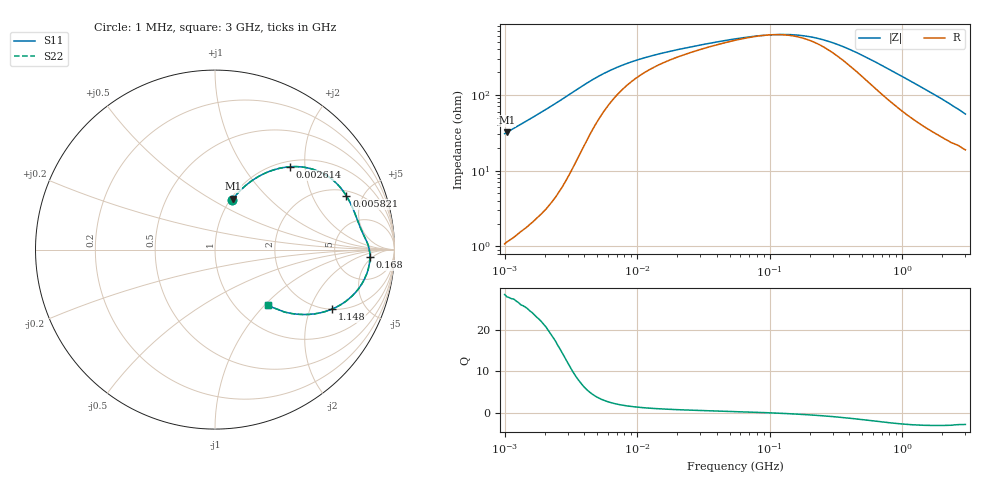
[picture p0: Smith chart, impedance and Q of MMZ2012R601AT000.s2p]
! S-parameter Generated by TDK Corporation
! Copyright(C) 2016 TDK Corporation.
! All Rights Reserved.
! TDK P/N: MMZ2012R601AT000 (Chip Beads)
! Property: |Z|=600¶ at 100MHz
! Size(LxWxT): 2x1.25x0.85mm, 0.079x0.049x0.033inches
! Model Type: s2p (Touchstone File Format Version 1.0)
! Frequency: DC=Yes Start=1MHz Stop=3000MHz 202points Log-sweep
! Note: This model was converted from impedance.
! Model Generated on May. 16, 2016
! Hash(MD5):
! Port Assignments:
!  1 ---@@@--- 2
! Applicable Conditions:
!  Temperature = 25 degC
!  DC Bias Current = 0 A
!  Small Signal Operation
! Terms and conditions regarding TDK Simulation Models
! (1)This simulation model is being provided solely for informational purposes. Please refer to the specifications of the products in terms of detailed characteristics of such products.
! (2)In no event shall TDK Corporation of any of its subsidiaries be liable for any loss or damage arising, directly or indirectly,
!  From any information contained in this simulation model, including, but not limited to loss or damages arising from any inaccuracies, omissions or errors in connection with such information.
! (3)Any and all copyrights on this simulation model are owned by TDK Corporation.
!  Duplication or redistribution of this simulation model without prior written permission from TDK Corporation is prohibited.
! (4)This simulation model is subject to any modification or change without any prior notice.
! (5)Neither TDK Corporation nor any of its subsidiaries shall make any warranty, express or implied,
!  Including but not limited to the correctness, implied warranties of merchantability and fitness for a particular purpose with respect to this simulation models.
! (6)The use of this simulation model shall be deemed to have consented to the terms and conditions hereof.
# MHz S MA R 50
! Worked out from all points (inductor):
!   201 points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, 1 MHz to 3 GHz, reference 50 ohm
!   read as one part in series: L = 4.88 uH near 1.041 MHz
!   highest Q = 27.9 at 1.041 MHz (marker M1), where L = 4.87 uH
!   self-resonance near 99.71 MHz
!   S11 on the Smith chart (normalised r, x): 1 MHz: 1.02, +0.61; 2.614 MHz: 1.11, +1.67; 5.821 MHz: 2.32, +3.71; 168 MHz: 12, -4; 1.148 GHz: 2.01, -2.87; 3 GHz: 1.37, -1.05
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1  0.2901 71.1  0.9468 -16.9  0.9468 -16.9  0.2901 71.1
1.040844  0.3008 70.4  0.943 -17.5  0.943 -17.5  0.3008 70.4
1.323425  0.3715 66.0  0.9142 -21.8  0.9142 -21.8  0.3715 66.0
1.682724  0.4535 60.6  0.8722 -26.9  0.8722 -26.9  0.4535 60.6
2.613693  0.6212 48.0  0.7444 -38.3  0.7444 -38.3  0.6212 48.0
3.19288  0.6916 41.0  0.6594 -43.5  0.6594 -43.5  0.6916 41.0
3.900413  0.7441 33.9  0.5647 -47.3  0.5647 -47.3  0.7441 33.9
4.764734  0.7753 27.5  0.475 -48.9  0.475 -48.9  0.7753 27.5
5.820586  0.7908 22.2  0.4019 -48.2  0.4019 -48.2  0.7908 22.2
9.040831  0.8052 14.4  0.2977 -42.3  0.2977 -42.3  0.8052 14.4
14.61624  0.8163 9.5  0.2366 -34.5  0.2366 -34.5  0.8163 9.5
54.77226  0.8493 2.6  0.1561 -14.0  0.1561 -14.0  0.8493 2.6
103.9275  0.8606 -0.2  0.1395 1.2  0.1395 1.2  0.8606 -0.2
168.0187  0.8644 -2.7  0.1425 16.6  0.1425 16.6  0.8644 -2.7
213.6344  0.8645 -4.2  0.1519 24.8  0.1519 24.8  0.8645 -4.2
306.2963  0.861 -7.1  0.1804 36.2  0.1804 36.2  0.861 -7.1
457.0858  0.8479 -11.4  0.2376 44.7  0.2376 44.7  0.8479 -11.4
800.5644  0.7966 -20.0  0.3702 47.3  0.3702 47.3  0.7966 -20.0
1147.801  0.7316 -26.9  0.4803 43.6  0.4803 43.6  0.7316 -26.9
1855.641  0.5998 -37.0  0.6342 34.7  0.6342 34.7  0.5998 -37.0
2359.433  0.5172 -42.1  0.7073 29.4  0.7073 29.4  0.5172 -42.1
3000  0.428 -46.5  0.7708 23.8  0.7708 23.8  0.428 -46.5
